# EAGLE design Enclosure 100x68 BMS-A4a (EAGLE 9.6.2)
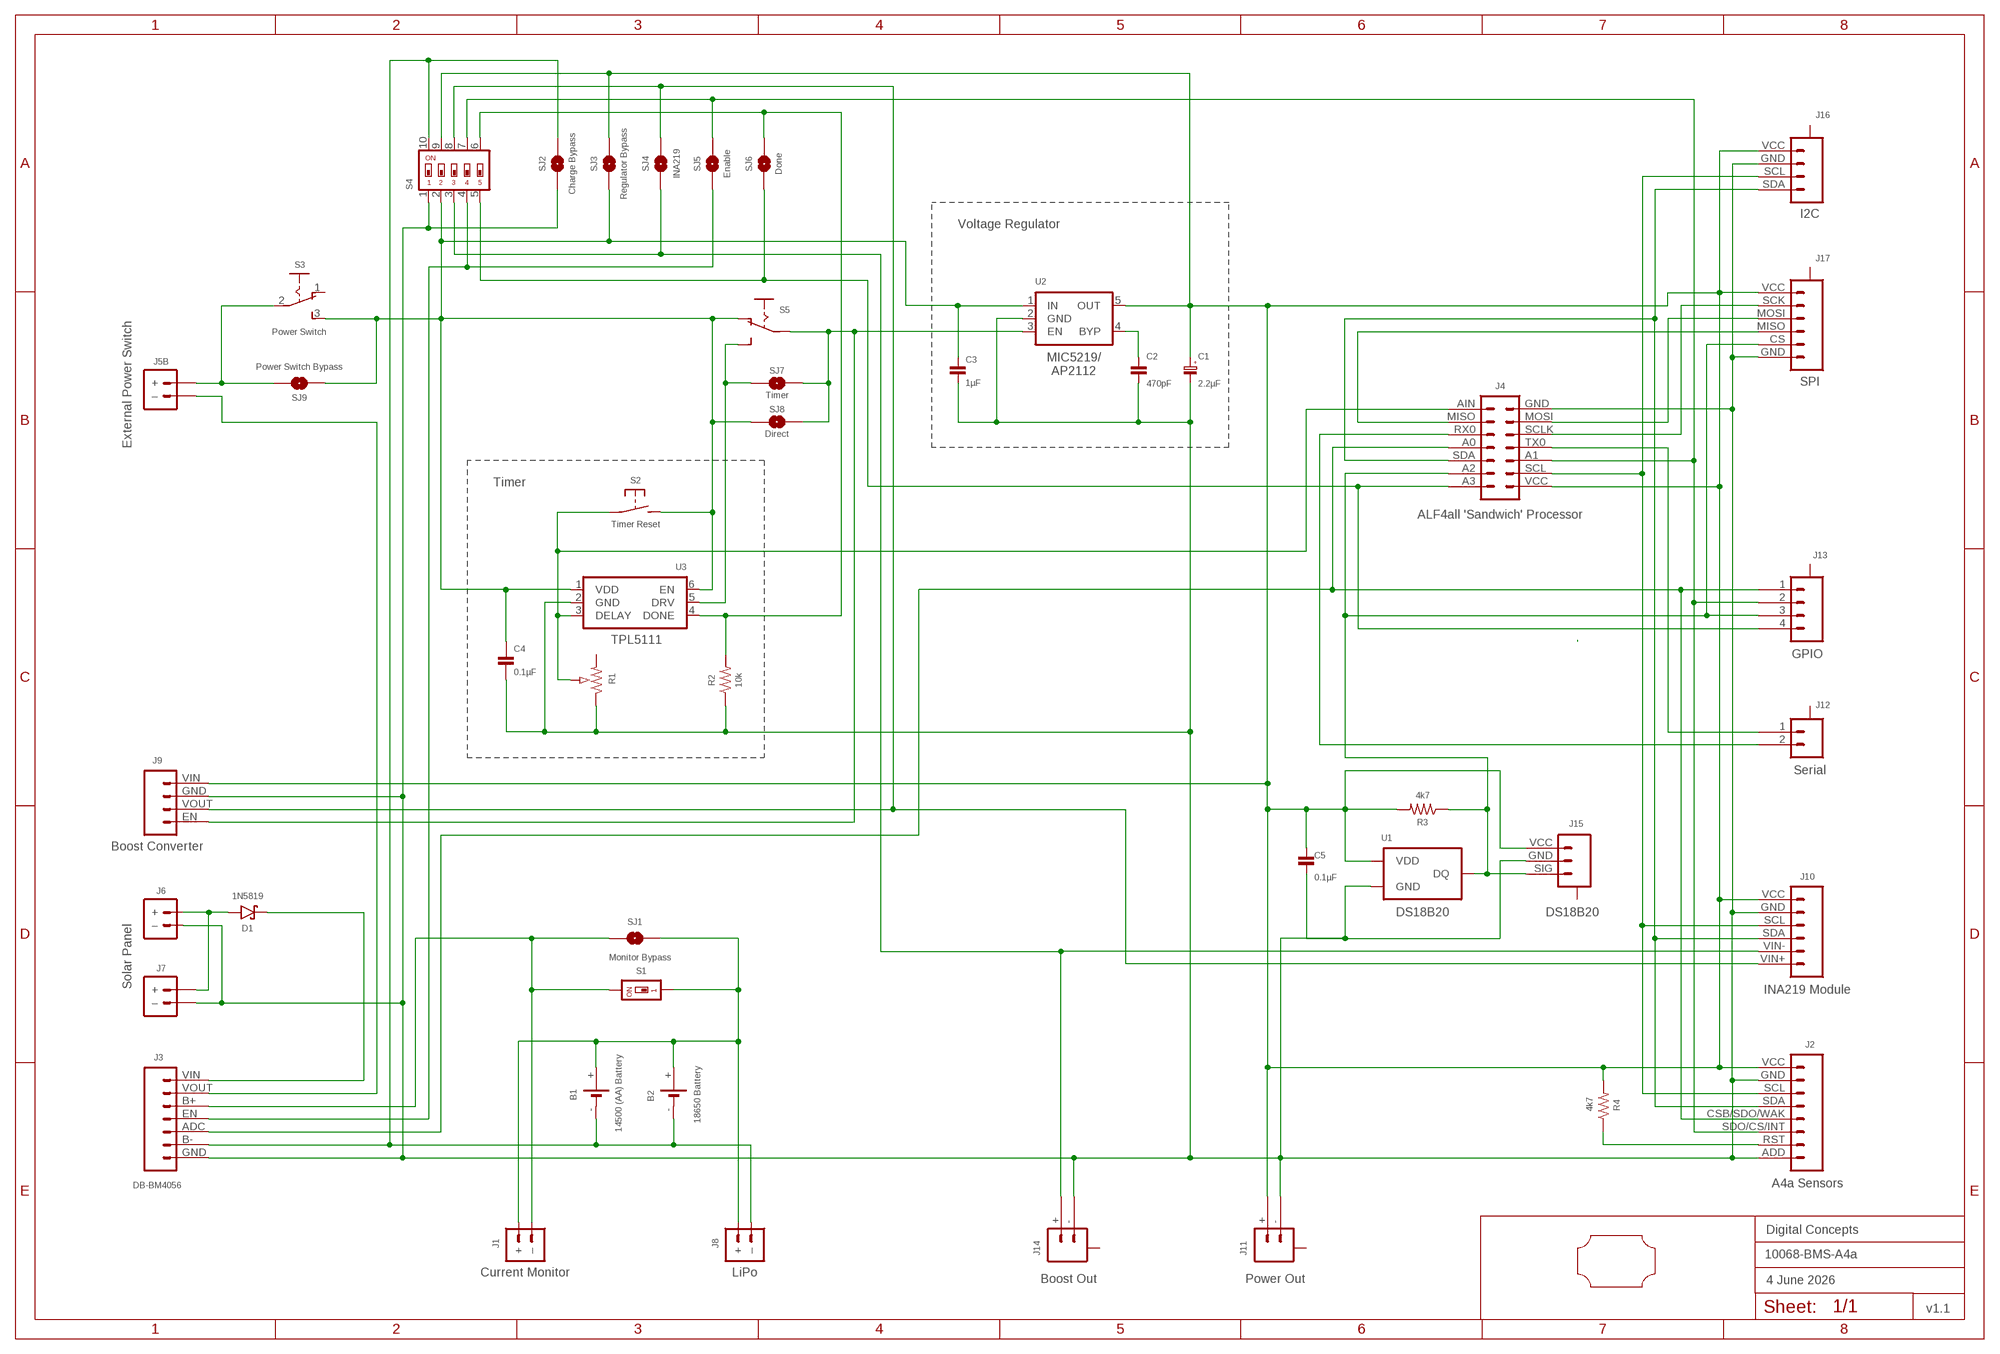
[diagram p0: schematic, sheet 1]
FRAME2 (A3L-LOC): DATE: 4 June 2026; OWNER: Digital Concepts; TITLE: 10068-BMS-A4a; VERSION: v1.1

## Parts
B1  14500 (AA) Battery  BATTERY-HOLDER-14500(AA)  [BATTERY-14500]
B2  18650 Battery  BATTERY-HOLDER-18650  [BATTERY-18650]
C1  2.2µF  CAPACITOR-1206-TANTALUM  [C1206-POLARISED]
C2  470pF  CAPACITOR-0805  [C0805]
C3  1µF  CAPACITOR-0805  [C0805]
C4  0.1µF  CAPACITOR  [C0805@1]
C5  0.1µF  CAPACITOR-0805  [C0805]
D1  1N5819  DIODE-SCHOTTKY-1N5819  [SOD-123]
J1  Current Monitor  JST-PH2.0-2-MALE-HORIZONTALJST-PTH-2  [JST-PH2.0-2-HORIZONTAL]
J2  A4a Sensors  HEADER-1X8-SENSOR  [CONN_08-SENSOR]
J3  DB-BM4056  HEADER-1X7-BCS  [CONN_07-BCS]
J4  ALF4all 'Sandwich' Processor  ALF4ALL-PROCESSOR-BOARD  [ALF4ALL-PROCESSOR-BOARD]
J5B  External Power Switch  JST-PH2.0-2-DUAL-POWERJST-PTH-2  [JST-PH2.0-2-DUAL-POWER]
J6  Solar Panel  JST-PH2.0-2-VERTICAL  [JST-PH2.0-2-VERTICAL=POWER]
J7  JST-PH2.0-2-HORIZONTAL-POWERJST-PTH-2  [JST-PH2.0-2-HORIZONTAL-POWER@1]
J8  LiPo  JST-PH2.0-2-MALE-HORIZONTALJST-PTH-2  [JST-PH2.0-2-HORIZONTAL]
J9  Boost Converter  HEADER-1X4-BOOST  [CONN_04-BOOST]
J10  INA219 Module  INA219-I2C-MODULE  [CONN_06-INA219]
J11  Power Out  JST-SH1.0-2-SMD-HORIZONTAL-POWER  [JST-SH1.0-2-SMD-HORIZONTAL-POWER]
J12  Serial  JST-SH1.0-2-SMD-HORIZONTAL  [JST-SH1.0-2-SMD-HORIZONTAL]
J13  GPIO  JST-SH1.0-4-SMD-HORIZONTAL  [JST-SH1.0-4-SMD-HORIZONTAL]
J14  Boost Out  JST-SH1.0-2-SMD-HORIZONTAL-POWER  [JST-SH1.0-2-SMD-HORIZONTAL-POWER]
J15  DS18B20  JST-SH1.0-3-SMD-HORIZONTAL-SIG  [JST-SH1.0-3-SMD-HORIZONTAL-SIG]
J16  I2C  JST-SH1.0-4-SMD-HORIZONTAL-I2C  [JST-SH1.0-4-SMD-HORIZONTAL-I2C]
J17  SPI  JST-SH1.0-6-SMD-HORIZONTAL-SPI  [JST-SH1.0-6-SMD-HORIZONTAL-SPI]
R1  RESISTOR-TRIMM-BAOTER-V-US  [RTRIM3296]
R2  10k  RESISTORR0805  [R0805]
R3  4k7  RESISTORR0805  [R0805]
R4  4k7  RESISTORR0805  [R0805]
S1  Monitor Bypass  SWITCH-DIP-SWS001-VIA-1  [SMD-001-VIA-1]
S2  Timer Reset  SWITCH-MOMENTARY-2-PIN-VIA-1  [SWITCH-2-PAD-VIA-1]
S3  Power Switch  SWITCH-SLIDE-SPDT  [SWITCH-SPDT-PTH]
S4  SWITCH-DIP-SWS005  [SMD-005]
S5  SWITCH-SLIDE-SPDT-SMT  [SWITCH-SPDT-SMT]
SJ1  Monitor Bypass  SJ  [SJ]
SJ2  Charge Bypass  SJ  [SJ]
SJ3  Regulator Bypass  SJ-V-12  [SJ-VIA-12]
SJ4  INA219  SJ  [SJ]
SJ5  Enable  SJ-V-1  [SJ-VIA-1]
SJ6  Done  SJ-V-1  [SJ-VIA-1]
SJ7  Timer  SJ-V-2  [SJ-VIA-2]
SJ8  Direct  SJ  [SJ]
SJ9  Power Switch Bypass  SJ  [SJ]
U1  DS18B20  THERMOMETER-DS18B20  [TO-92]
U2  MIC5219  [SOT-23-5]
U3  TPL5111  TPL5111DDCR  [SOT-23-6]
U$1  PCB-OUTLINE-100X68-CUT  [PROTO-34X22-OUTLINE-CUT]

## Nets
A0: J2.CSB/SDO/WAK J3.ADC J4.A0 J13.1
A1: J2.SDO/CS/INT J4.A1 J13.2 S4.7 SJ5.1 SJ5.1@V
A2: J4.A2 J13.3 J15.SIG J17.CS R3.1 U1.2(DQ)
A3: J4.A3 J13.4 S4.5 SJ6.2
AIN: J4.AIN R1.2(S) S2.1(P) S2.1@VIA(P) U3.3(DELAY)
B+: B1.+ B2.+ J1.+ J8.+ S1.1 S1.1@VIA SJ1.1
B-: B1.- B2.- J3.B- J8.-(–) S4.10 SJ2.2
BOOST-VOUT: J9.VOUT J10.VIN+ S4.8 SJ4.2
CHARGE-VOUT: J3.VOUT J5B.-(–)
GND: C1.2(-) C2.2 C3.2 C4.1 C5.2 J2.ADD J2.GND J3.GND J4.GND J6.-(–) J7.-(–) J9.GND J10.GND J11.- J14.- J15.GND J16.GND J17.GND R1.1(A) R2.1 S4.1 SJ2.1 U1.1(GND) U2.2(GND) U3.2(GND)
I-B+: J1.-(–) J3.B+ S1.2 SJ1.2
MISO: J4.MISO J17.MISO
MOSI: J4.MOSI J17.MOSI
N$1: C3.1 C4.2 S2.2(S) S3.3(S) S4.2 S5.1(O) SJ3.2 SJ3.2@V SJ8.2 SJ9.1 U2.1(IN) U3.1(VDD) U3.6(EN)
N$2: J9.EN S5.2(P) SJ7.1 SJ8.1 U2.3(EN)
N$3: C2.1 U2.4(BYP)
N$4: R2.2 S4.6 SJ6.1 SJ6.1@V U3.4(DONE)
N$5: J3.EN S4.4 SJ5.2
N$6: J5B.+ S3.2(P) SJ9.2
N$7: D1.A J6.+ J7.+
N$8: D1.C J3.VIN
N$9: S5.3(S) SJ7.2 SJ7.2@V U3.5(DRV)
RST: J2.RST R4.1
RXO: J4.RX0 J12.2
SCK: J4.SCLK J17.SCK
SCL: J2.SCL J4.SCL J10.SCL J16.SCL
SDA: J2.SDA J4.SDA J10.SDA J16.SDA
TXO: J4.TX0 J12.1
VCC: C1.1(+) C5.1 J2.VCC J4.VCC J9.VIN J10.VCC J11.+ J15.VCC J16.VCC J17.VCC R3.2 R4.2 S4.9 SJ3.1 SJ3.1@V U1.3(VDD) U2.5(OUT)
VDD: J10.VIN- J14.+ S4.3 SJ4.1
Unconnected: J11.A@1(A) J11.A@2(A) J12.A@1(A) J12.A@2(A) J13.A@1(A) J13.A@4(A) J14.A@1(A) J14.A@2(A) J15.A@1(A) J15.A@3(A) J16.A@1(A) J16.A@4(A) J17.A@1(A) J17.A@6(A) R1.3(E) S3.1(O)

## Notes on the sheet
- Voltage Regulator
- MIC5219/
  AP2112
- Timer

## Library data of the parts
B1 = digitalconcepts:BATTERY-HOLDER-14500(AA): 14500 (AA) battery holder
B2 = digitalconcepts:BATTERY-HOLDER-18650: 18650 Battery Holder
C1 = digitalconcepts:CAPACITOR-1206-TANTALUM: Capacitor 1206 Tantalum
C2 C3 C5 = digitalconcepts:CAPACITOR-0805: 0805 Capacitor
C4 = digitalconcepts:CAPACITOR: 0805 Capacitor
D1 = digitalconcepts:DIODE-SCHOTTKY-1N5819: 1N5819 Schottky Diode SOD-123
J1 J8 = digitalconcepts:JST-PH2.0-2-MALE-HORIZONTAL: PH2.0 2P Right Angle PCB Connector; PROD_ID: CONN-09863; SKU: PRT-09914
J2 = digitalconcepts:HEADER-1X8-SENSOR: IoT Sensors 1x8 Pin Header for 'Sandwich' IoT Sensors
J3 = digitalconcepts:HEADER-1X7-BCS: Single Row 7-Pin Header BCS Pin labels
J4 = digitalconcepts:ALF4ALL-PROCESSOR-BOARD: ALF4all 'Sandwixh' Processor 2x7 Pin Header and earthed 1x1 locator pins for ALF4all 'Sandwich' Processor/RFM95W PCBs
J5B = digitalconcepts:JST-PH2.0-2-DUAL-POWER: JST PH2.0 2P PTH Dual-Side Connector (Power); PROD_ID: CONN-09863; SKU: PRT-09914
J6 = digitalconcepts:JST-PH2.0-2-VERTICAL: PH2.0 2P PCB Connector
J7 = digitalconcepts:JST-PH2.0-2-HORIZONTAL-POWER: PH2.0 2P Right Angle PCB Connector; PROD_ID: CONN-09863; SKU: PRT-09914
J9 = digitalconcepts:HEADER-1X4-BOOST: Boost Converter Module 4-Pin Header
J10 = digitalconcepts:INA219-I2C-MODULE: INA219 I2C Module
J11 J14 = digitalconcepts:JST-SH1.0-2-SMD-HORIZONTAL-POWER: JST SH1.0 2P SMD Horizontal Connector with Power Labels
J12 = digitalconcepts:JST-SH1.0-2-SMD-HORIZONTAL: JST SH1.0 2P SMD Horizontal Connector
J13 = digitalconcepts:JST-SH1.0-4-SMD-HORIZONTAL: JST SH1.0 4P SMD horizontal connector
J15 = digitalconcepts:JST-SH1.0-3-SMD-HORIZONTAL-SIG: JST SH1.0 3P SMD Horizontal Connector with Signal
J16 = digitalconcepts:JST-SH1.0-4-SMD-HORIZONTAL-I2C: JST SH1.0 4P SMD I2C horizontal connector
J17 = digitalconcepts:JST-SH1.0-6-SMD-HORIZONTAL-SPI: JST SH1.0 6P SMD SPI horizontal connector
R1 = digitalconcepts:RESISTOR-TRIMM-BAOTER-V-US: Trimm Resistor - Vertical BAOTER
R2-R4 = digitalconcepts:RESISTOR: Resistor; SPICEPREFIX: R
S1 = digitalconcepts:SWITCH-DIP-SWS001-VIA-1: SMD Dip Switch 1 pol.
S2 = digitalconcepts:SWITCH-MOMENTARY-2-PIN-VIA-1: 2 Pin Momentary Switch
S3 = digitalconcepts:SWITCH-SLIDE-SPDT: Mini Sliding Switch SPDT
S4 = digitalconcepts:SWITCH-DIP-SWS005: SMD Dip Switch 5 pol.
S5 = digitalconcepts:SWITCH-SLIDE-SPDT-SMT: Mini Sliding Switch SPDT SMT
SJ1 SJ2 SJ4 SJ8 SJ9 = digitalconcepts:SJ: Solder Jumper
SJ3 = digitalconcepts:SJ-V-12: Solder Jumper with Pad Vias
SJ5 SJ6 = digitalconcepts:SJ-V-1: Solder Jumper with single Pad Via
SJ7 = digitalconcepts:SJ-V-2: Solder Jumper with Pad Vias
U1 = digitalconcepts:THERMOMETER-DS18B20: Digital Thermometer -55C-125C TO92-3; AVAILABILITY: Bad; DESCRIPTION: Temperature Sensor Digital, Local -55°C ~ 125°C 12 b 8-uMAX; MF: Maxim Integrated; MP: DS18B20; PACKAGE: TO-92 Maxim Integrated; PRICE: None
U2 = digitalconcepts:MIC5219: Microchip LDO Linear Voltage Regulator; OC_FARNELL: unknown; OC_NEWARK: unknown
U3 = digitalconcepts:TPL5111DDCR: TPL5111 Nano-Power System Timer
U$1 = digitalconcepts:PCB-OUTLINE-100X68-CUT: PCB outline for 100 x 68 enclosure with long side cut-out

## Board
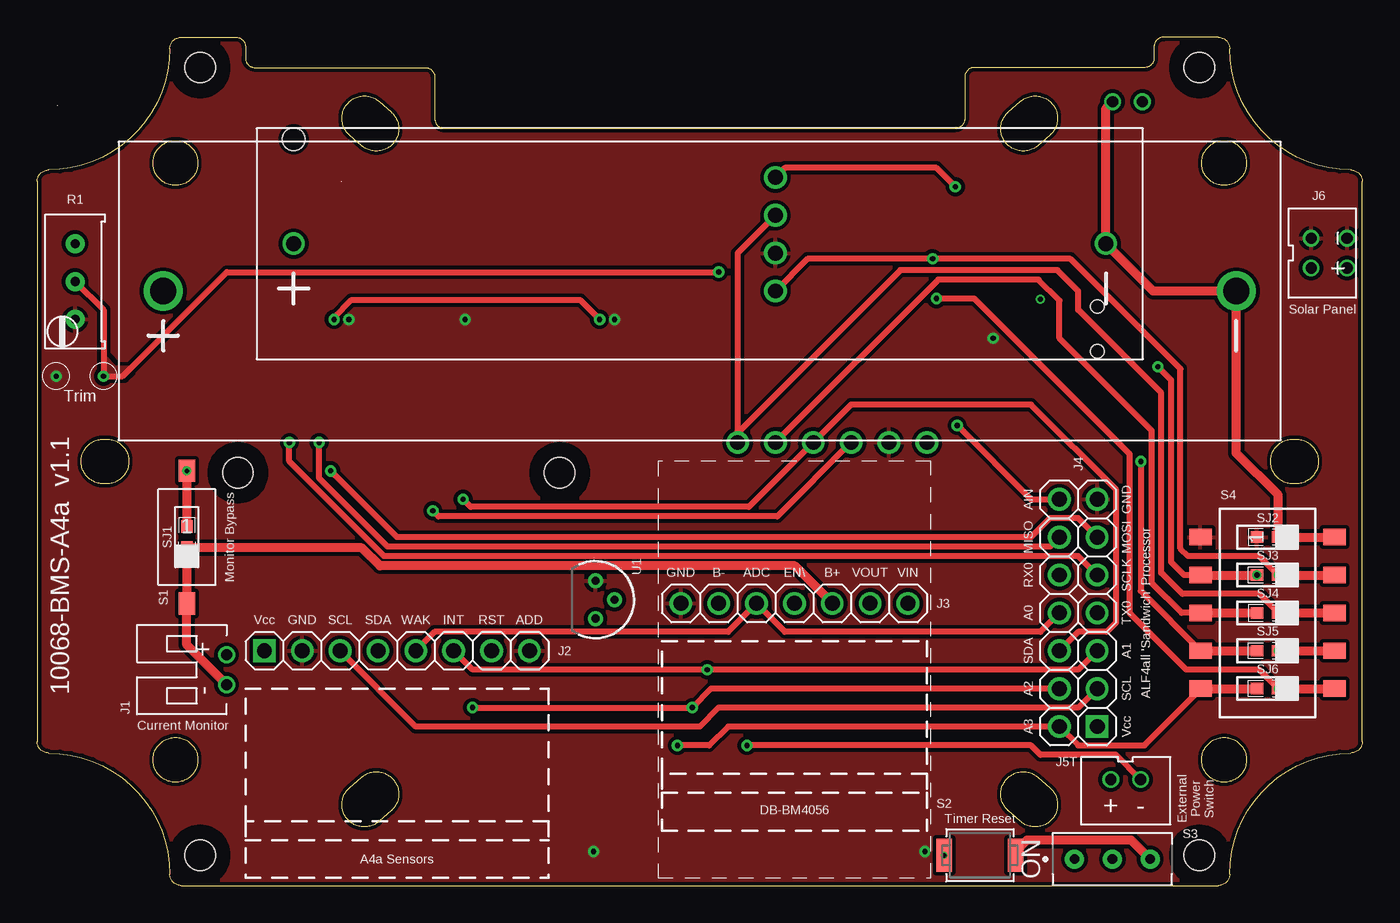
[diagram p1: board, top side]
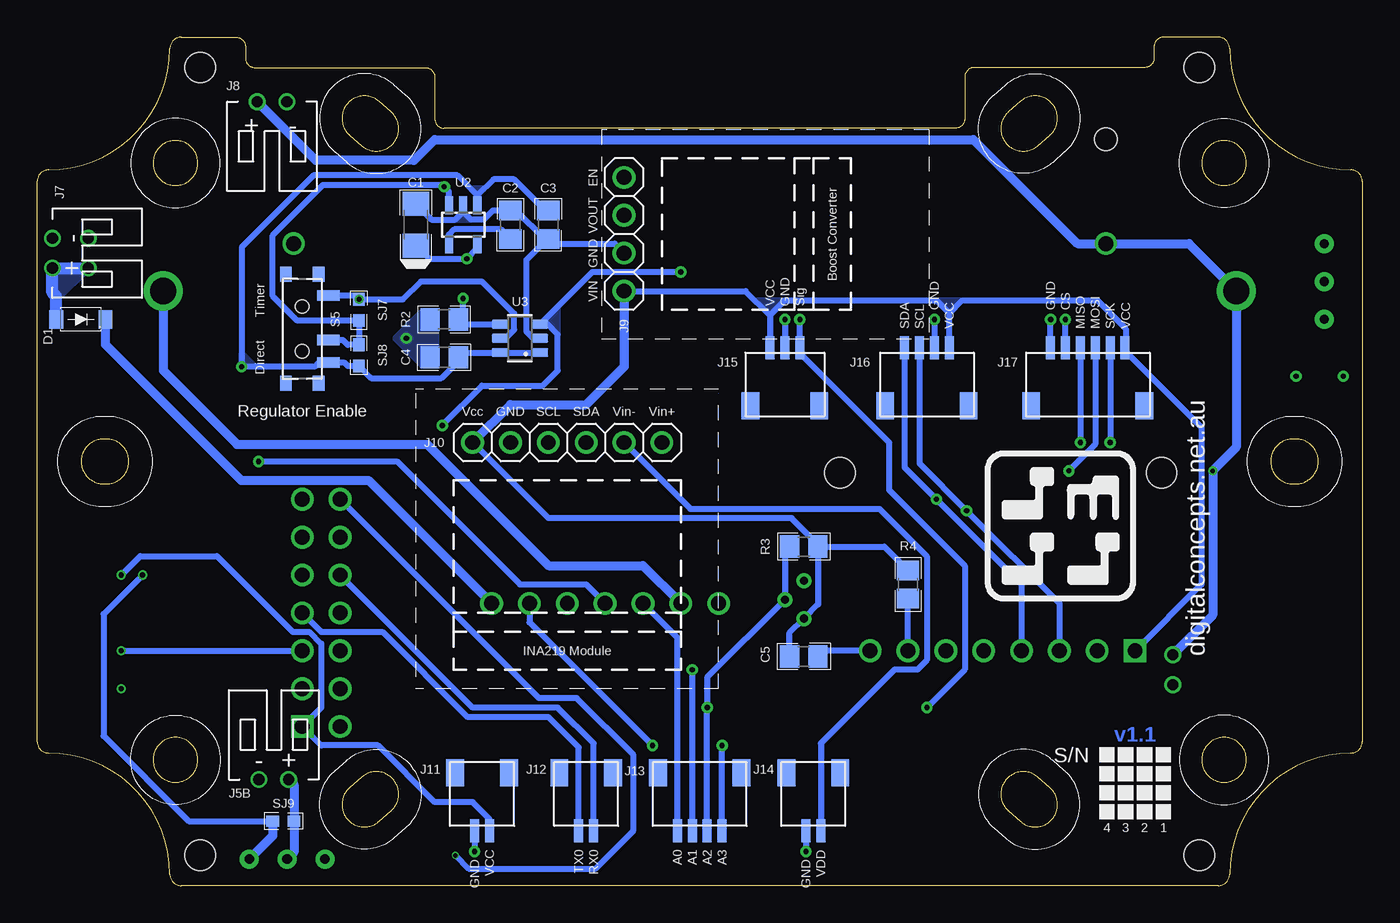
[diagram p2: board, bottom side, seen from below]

Size 88.9 x 56.9 mm. Coordinates in mm from the lower left corner, seen from the top.
Copper layers (1*16): Top 0.035mm / dielectric 1.5mm / Bottom 0.035mm
Design rules "default *": minimum track width 6mil, minimum drill 0.3mm, track to track 6mil, track to pad 6mil, pad to pad 6mil, via to via 6mil, smd to smd 6mil, copper to edge 6mil, drill to drill 6mil, minimum pad ring 1mil, minimum via ring 8mil, stop-mask expansion 4mil, vias tented up to drill 0mil, thermal gap 10mil
Holes 2.03 mm at 13.46,27.69 35.05,27.69

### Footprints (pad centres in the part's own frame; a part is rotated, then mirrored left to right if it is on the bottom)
BATTERY-14500 = drill 1: + -27.25,0; - 27.25,0 | hole 1.524: -27.25,7
BATTERY-18650 = drill 1.75: + -36,0; - 36,0
C1206-POLARISED = smd 1.6 x 1.8: 1 -1.4,0; 2 1.4,0
C0805 = smd 1.3 x 1.5: 1 -0.95,0; 2 0.95,0
C0805@1 = smd 1.3 x 1.5: 1 -0.95,0; 2 0.95,0
SOD-123 = smd 0.91 x 1.22: A -1.65,0; C 1.65,0
JST-PH2.0-2-HORIZONTAL = drill 0.75: + 1,0; - -1,0
CONN_08-SENSOR = drill 1 pad 1.524: ADD 17.78,0; CSB/SDO/WAK 10.16,0; GND 2.54,0; RST 15.24,0; SCL 5.08,0; SDA 7.62,0; SDO/CS/INT 12.7,0 | drill 1 pad 1.524 square: VCC 0,0
CONN_07-BCS = drill 1 pad 1.524: ADC 5.08,0; B+ 10.16,0; B- 2.54,0; EN 7.62,0; GND 0,0; VIN 15.24,0; VOUT 12.7,0
ALF4ALL-PROCESSOR-BOARD = drill 1 pad 1.524: A0 7.62,2.54; A1 5.08,0; A2 2.54,2.54; A3 0,2.54; AIN 15.24,2.54; GND 15.24,0; MISO 12.7,2.54; MOSI 12.7,0; RX0 10.16,2.54; SCL 2.54,0; SCLK 10.16,0; SDA 5.08,2.54; TX0 7.62,0 | drill 1 pad 1.524 square: VCC 0,0
JST-PH2.0-2-DUAL-POWER = drill 0.75: + 1,0; - -1,0
JST-PH2.0-2-VERTICAL=POWER = drill 0.75: + -1,0; - 1,0
JST-PH2.0-2-HORIZONTAL-POWER@1 = drill 0.75: + 1,0; - -1,0
CONN_04-BOOST = drill 1 pad 1.524: EN 0,0; GND 5.08,0; VIN 7.62,0; VOUT 2.54,0
CONN_06-INA219 = drill 1 pad 1.524: GND 2.54,0; SCL 5.08,0; SDA 7.62,0; VCC 0,0; VIN+ 12.7,0; VIN- 10.16,0
JST-SH1.0-2-SMD-HORIZONTAL-POWER = smd 0.6 x 1.55: + -0.5,2.54; - 0.5,2.54 | smd 1.2 x 1.8: A@1 1.8,-1.335; A@2 -1.8,-1.335
JST-SH1.0-2-SMD-HORIZONTAL = smd 0.6 x 1.55: 1 0.5,2.54; 2 -0.5,2.54 | smd 1.2 x 1.8: A@1 1.8,-1.335; A@2 -1.8,-1.335
JST-SH1.0-4-SMD-HORIZONTAL = smd 0.6 x 1.55: 1 1.5,2.54; 2 0.5,2.54; 3 -0.5,2.54; 4 -1.5,2.54 | smd 1.2 x 1.8: A@1 2.8,-1.335; A@4 -2.8,-1.335
JST-SH1.0-3-SMD-HORIZONTAL-SIG = smd 1.2 x 1.8: A@1 2.3,-1.335; A@3 -2.3,-1.335 | smd 0.6 x 1.55: GND 0,2.54; SIG 1,2.54; VCC -1,2.54
JST-SH1.0-4-SMD-HORIZONTAL-I2C = smd 1.2 x 1.8: A@1 2.8,-1.335; A@4 -2.8,-1.335 | smd 0.6 x 1.55: GND 0.5,2.54; SCL -0.5,2.54; SDA -1.5,2.54; VCC 1.5,2.54
JST-SH1.0-6-SMD-HORIZONTAL-SPI = smd 1.2 x 1.8: A@1 3.8,-1.335; A@6 -3.8,-1.335 | smd 0.6 x 1.55: CS -1.5,2.54; GND -2.5,2.54; MISO -0.5,2.54; MOSI 0.5,2.54; SCK 1.5,2.54; VCC 2.5,2.54
RTRIM3296 = drill 0.61 pad 1.27: 1 0,-2.54; 2 0,0; 3 0,2.54
R0805 = smd 1.3 x 1.5: 1 -0.95,0; 2 0.95,0
SMD-001-VIA-1 = smd 1.1 x 1.5: 1 0,-4.45; 2 0,4.45 | drill 0.3 pad 0.61: 1@VIA 0,-4.45
SWITCH-2-PAD-VIA-1 = smd 1.067 x 2.184: 1 -2.4,0; 2 2.4,0 | drill 0.3: 1@VIA -2.4,0
SWITCH-SPDT-PTH = drill 0.65 pad 1.27: 1 -2.54,0; 2 0,0; 3 2.54,0
SMD-005 = smd 1.1 x 1.5: 1 -5.08,-4.5; 2 -2.54,-4.5; 3 0,-4.5; 4 2.54,-4.5; 5 5.08,-4.5; 6 5.08,4.5; 7 2.54,4.5; 8 0,4.5; 9 -2.54,4.5; 10 -5.08,4.5
SWITCH-SPDT-SMT = smd 0.7 x 1.5: 1 2.25,1.75; 2 0.75,1.75; 3 -2.25,1.75 | smd 1 x 0.8: GND@1 3.65,-1.1; GND@2 3.65,1.1; GND@3 -3.65,1.1; GND@4 -3.65,-1.1 | hole 0.9: -1.5,0; 1.5,0
SJ = smd 0.864 x 0.762: 1 -0.711,0; 2 0.711,0
SJ-VIA-12 = smd 0.864 x 0.762: 1 -0.711,0; 2 0.711,0 | drill 0.35 pad 0.61: 1@V -0.711,0; 2@V 0.711,0
SJ-VIA-1 = smd 0.864 x 0.762: 1 -0.711,0; 2 0.711,0 | drill 0.35 pad 0.61: 1@V -0.711,0
SJ-VIA-2 = smd 0.864 x 0.762: 1 -0.711,0; 2 0.711,0 | drill 0.35 pad 0.61: 2@V 0.711,0
TO-92 = drill 0.55 pad 1.016: 1 -1.27,0; 2 0,1.27; 3 1.27,0
SOT-23-5 = smd 0.55 x 1.2: 1 -0.95,-1.3; 2 0,-1.3; 3 0.95,-1.3; 4 0.95,1.3; 5 -0.95,1.3
SOT-23-6 = smd 1.1 x 0.6: 1 -1.35,0.95; 2 -1.35,0; 3 -1.35,-0.95; 4 1.35,-0.95; 5 1.35,0; 6 1.35,0.95
PROTO-34X22-OUTLINE-CUT = hole 2.032: -33.528,26.416; 33.528,26.416; 33.528,-26.416; -33.528,-26.416

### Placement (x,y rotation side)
B1  44.45,43.05 0 top
B2  44.45,39.88 0 top
C1  63.5,44.32 90 bottom
C2  57.15,44.32 90 bottom
C3  54.61,44.32 270 bottom
C4  61.59,35.43 0 bottom
C5  37.47,15.37 0 bottom
D1  85.98,37.97 0 bottom
J1  12.7,14.48 90 top
J2  15.24,15.75 0 top
J3  43.18,18.92 0 top
J4  71.12,10.67 90 top
J5B  73.03,7.11 0 bottom
J6  85.47,42.42 90 top
J7  87.88,42.42 270 bottom
J8  73.15,52.58 180 bottom
J9  49.53,47.5 270 bottom
J10  59.69,29.72 0 bottom
J11  59.06,6.22 180 bottom
J12  52.07,6.22 180 bottom
J13  44.45,6.22 180 bottom
J14  36.83,6.22 180 bottom
J15  38.73,33.53 0 bottom
J16  29.21,33.53 0 bottom
J17  18.42,33.53 0 bottom
R1  2.54,40.51 0 top
R2  61.59,37.97 0 bottom
R3  37.47,22.73 0 bottom
R4  30.48,20.19 90 bottom
S1  10.03,23.37 180 top
S2  63.25,2.03 0 top
S3  72.14,1.78 0 top
S4  82.55,18.29 270 top
S5  71.12,37.34 270 bottom
SJ1  10.03,23.37 270 top
SJ2  82.55,23.37 0 top
SJ3  82.55,20.83 180 top
SJ4  82.55,18.29 0 top
SJ5  82.55,15.75 180 top
SJ6  82.55,13.21 180 top
SJ7  67.31,38.61 90 bottom
SJ8  67.31,35.56 270 bottom
SJ9  72.39,4.32 0 bottom
U1  37.47,19.18 270 top
U2  60.33,44.32 180 bottom
U3  56.52,36.7 180 bottom
U$1  44.45,28.45 0 top

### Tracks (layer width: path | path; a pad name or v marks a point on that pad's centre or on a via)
$X0
  cutout Bottom: 10.92,56.9 arc180 10.92,52.83 arc180
$X1
  cutout Bottom: 77.98,56.9 arc180 77.98,52.83 arc180
$X2
  cutout Bottom: 77.98,4.06 arc180 77.98,0 arc180
$X3
  cutout Bottom: 10.92,4.06 arc180 10.92,0 arc180
$X4
  cutout Top: 10.92,56.9 arc180 10.92,52.83 arc180
$X5
  cutout Top: 77.98,56.9 arc180 77.98,52.83 arc180
$X6
  cutout Top: 77.98,4.06 arc180 77.98,0 arc180
$X7
  cutout Top: 10.92,4.06 arc180 10.92,0 arc180
$X8
  cutout Bottom: 13.46,29.72 arc180 13.46,25.65 arc180
$X9
  cutout Top: 35.05,29.72 arc180 35.05,25.65 arc180
$X10
  cutout Top: 13.46,29.72 arc180 13.46,25.65 arc180
$X11
  cutout Bottom: 35.05,29.72 arc180 35.05,25.65 arc180
A0
  Top 0.406: J4.A0 67.31,17.02 50.16,17.02 J3.ADC 46.36,17.02 26.67,17.02 J2.CSB/SDO/WAK
  Bottom 0.406: J3.ADC 45.95,16.61 J13.1
A1  (via drill 0.35)
  Top 0.406: J4.A1 69.85,14.48 v44.95,14.48 29.21,14.48 J2.SDO/CS/INT
  Top 0.61: SJ5.1@V S4.7
  Bottom 0.406: SJ5.1@V J4.A1 | J13.2 v44.95,14.48
A2  (via drill 0.35)
  Top 0.406: J4.A2 45.22,13.21 v43.95,11.94 v29.21,11.94 | v37.73,37.97 36.47,39.24 21.06,39.24 19.92,38.1 v19.92,37.97
  Bottom 0.406: R3.1 38.73,22.41 U1.2 43.95,13.96 v43.95,11.94 J13.3 | J17.CS v19.92,37.97 | v37.73,37.97 J15.SIG 37.73,35.7 31.75,29.72 31.75,26.54 26.67,21.46 26.67,14.48 v29.21,11.94
A3  (via drill 0.35)
  Top 0.406: v42.95,9.4 45.09,9.4 46.36,10.67 J4.A3 69.85,9.4 74.3,9.4 78.05,13.15 S4.5
  Top 0.61: S4.5 SJ6.2
  Bottom 0.406: J13.4 v42.95,9.4
AIN  (via drill 0.35)
  Top 0.406: J4.AIN 66.67,25.91 v61.72,30.86 | R1.2 4.45,38.61 v4.45,34.16 5.73,34.16 12.71,41.15 v45.72,41.15
  Bottom 0.406: v61.72,30.86 59.06,33.53 54.99,33.53 53.98,34.54 53.98,36.96 54.67,37.65 U3.3 51.67,41.15 v45.72,41.15 | S2.1@VIA 59.96,1.14 51.44,1.14 48.9,3.68 48.9,8.76 52.7,12.57 55.25,12.57 J4.AIN
  pour Bottom (no thermals): 54.86,37.85 53.98,38.73 53.98,36.96
  pour Top (no thermals): 4.45,34.16 5.72,34.16 6.22,34.67 5.21,34.67 4.45,35.43
B+
  Top 0.61: S1.1@VIA SJ1.1
  Bottom 0.61: J1.+ 10.03,18.15 S1.1@VIA 8.45,29.4 B2.+ 11.62,43.05 B1.+ 19.11,43.05 26.09,50.04 62.23,50.04 63.63,48.64 70.22,48.64 J8.+
B-
  Top 0.61: J8.- 71.7,52.13 B1.- 74.88,39.88 B2.- 80.45,29.01 83.26,26.2 SJ2.2 S4.10
  Bottom 0.61: B2.- 80.45,34.55 75.49,29.59 62.74,29.59 54.61,21.46 48.26,21.46 J3.B-
BOOST-VOUT
  Top 0.406: J9.VOUT 46.99,42.42 J10.VIN+ 46.99,30.35 57.91,41.28 68.45,41.28 69.85,39.88 69.85,38.61 75.41,33.05 75.41,20.98 76.84,19.56 81.99,19.56 SJ4.2
  Top 0.61: SJ4.2 S4.8
CHARGE-VOUT  (via drill 0.35)
  Top 0.406: J5B.- 72.39,8.75 72.39,8.76 67.31,8.76 66.67,9.4 v47.62,9.4
  Bottom 0.406: J3.VOUT 55.88,17.65 v47.62,9.4
GND  (via drill 0.35)
  Bottom 0.406: C1.2 62.45,44.67 60.85,44.67 60.33,45.2 | 60.33,45.2 59.8,44.67 58.95,44.67 58.35,45.27 C2.2 56.77,45.27 54.87,43.37 C3.2 54.61,43.31 54.36,43.05 | U2.2 60.33,45.2 | U3.2 55.63,36.7 56.08,37.16 56.08,41.96 54.99,43.05 54.36,43.05 | 54.36,43.05 50.16,43.05 J9.GND | v38.73,37.97 J15.GND | v28.71,37.97 J16.GND | J17.GND v20.92,37.97 | J14.- v37.33,2.29 | J11.- v59.56,2.29 | J2.ADD 36.13,15.75 C5.2
  other vias: 64.14,36.7 1.27,34.16
  pour Top (isolate 0.254, rank 5): -1.06,57.55 -1.06,-0.7 89.91,-0.7 89.91,57.55
  pour Bottom (no thermals): 60.33,45.2 60.85,44.67 59.8,44.67
  pour Bottom (no thermals): 64.9,36.7 63.12,34.93 62.1,34.93 62.1,38.48 63.12,38.48
I-B+
  Top 0.61: J1.- 10.03,16.15 S1.2 SJ1.2 21.77,22.66 22.99,21.44 50.83,21.44 J3.B+
MISO  (via drill 0.35)
  Top 0.406: J4.MISO 67.95,22.73 23.5,22.73 18.92,27.31 v18.92,29.72
  Bottom 0.406: J17.MISO v18.92,29.72
MOSI  (via drill 0.35)
  Top 0.406: J4.MOSI 69.85,24.64 67.95,24.64 66.67,23.37 24.13,23.37 v19.69,27.81
  Bottom 0.406: J17.MOSI 17.92,29.58 v19.69,27.81
N$1  (via drill 0.35)
  Top 0.406: S4.2 76.96,20.83 76.07,21.71 76.07,33.91 v75.18,34.8
  Top 0.61: S2.2 65.65,2.29 66.41,3.05 73.41,3.05 S3.3 | S4.2 SJ3.2@V
  Bottom 0.406: 59.38,46.29 58.3,47.37 56.9,47.37 54.8,45.27 C3.1 | 59.38,46.29 60.71,47.62 70.36,47.62 75.18,42.8 v75.18,34.8 70.3,34.8 70,35.09 S5.1 68.31,35.09 68.07,34.85 SJ8.2 66.5,34.04 61.78,34.04 60.64,35.18 C4.2 60.85,35.75 U3.6 U3.1 | 59.38,46.29 U2.1 | SJ3.2@V 84.45,18.21 84.45,10.03 78.74,4.32 SJ9.1
  Bottom 0.61: SJ9.1 73.1,3.35 S3.3
  pour Bottom (no thermals): 58.93,46.74 59.82,46.74 59.38,46.29
  pour Bottom (no thermals): 75.18,34.8 75.18,35.69 74.3,34.8
N$2  (via drill 0.35)
  Top 0.406: v61.59,46.86 60.33,48.13 50.16,48.13 J9.EN
  Bottom 0.406: U2.3 61.28,46.54 v61.59,46.86 61.72,46.99 69.72,46.99 73.1,43.61 73.1,39.54 71.46,37.9 SJ7.1 SJ8.1 68.07,36.27 68.39,36.59 S5.2
N$3
  Bottom 0.406: U2.4 61.28,43.66 60.92,44.01 57.79,44.01 C2.1
N$4  (via drill 0.35)
  Top 0.406: v60.33,39.37 62.86,39.37 73.28,28.96 73.28,18.29 77.09,14.48 81.99,14.48 SJ6.1@V
  Top 0.61: SJ6.1@V S4.6
  Bottom 0.406: U3.4 60.33,37.65 R2.2 60.33,38.29 v60.33,39.37
N$5  (via drill 0.35)
  Top 0.406: S4.4 74.04,19.76 v74.04,28.45
  Top 0.61: S4.4 SJ5.2
  Bottom 0.406: v74.04,28.45 64.77,28.45 56.52,20.19 52.07,20.19 J3.EN
N$6
  Bottom 0.61: J5B.+ 71.68,6.77 SJ9.2 71.68,2.24 S3.2
N$7
  Bottom 0.813: D1.A 87.63,39.51 87.88,39.77 J7.+ J6.+
  pour Bottom (no thermals): 87.63,41.42 85.73,41.42 87.63,39.51
N$8
  Bottom 0.61: D1.C 84.33,36.3 75.21,27.18 66.67,27.18 J3.VIN
N$9
  Bottom 0.406: U3.5 57.48,36.7 56.9,37.29 56.9,38.35 59.06,40.51 63.18,40.51 64.37,39.32 SJ7.2@V 67.58,39.59 S5.3
RST
  Bottom 0.406: J2.RST R4.1
RXO
  Bottom 0.406: J12.2 51.57,9.53 53.98,11.94 59.69,11.94 J4.RX0
SCK  (via drill 0.35)
  Top 0.406: J4.SCLK 69.85,22.1 23.27,22.1 16.92,28.45 v16.92,29.72
  Bottom 0.406: J17.SCK v16.92,29.72
SCL  (via drill 0.35)
  Top 0.406: J4.SCL 69.85,11.94 45.72,11.94 44.45,10.67 25.4,10.67 J2.SCL | J10.SCL 49.66,24.77 26.92,24.77 v26.54,25.15
  Bottom 0.406: J16.SCL 29.71,28.31 v26.54,25.15 20.32,18.92 J2.SCL
SDA  (via drill 0.35)
  Top 0.406: v28.58,25.91 29.08,25.4 47.75,25.4 J10.SDA 54.61,32.26 66.67,32.26 72.39,26.54 72.39,17.65 71.75,17.02 69.85,17.02 J4.SDA
  Bottom 0.406: J16.SDA 30.71,28.04 v28.58,25.91 22.86,20.19 J2.SDA
TXO
  Bottom 0.406: J12.1 52.57,9.26 54.61,11.3 60.01,11.3 65.73,17.02 69.85,17.02 J4.TX0
VCC  (via drill 0.35)
  Top 0.406: J9.VIN 51.69,42.04 v60.07,42.04 69.32,42.04 76.71,34.65 76.71,22.61 77.22,22.1 81.99,22.1 SJ3.1@V
  Top 0.61: SJ3.1@V S4.9
  Bottom 0.406: C1.1 62.61,42.04 v60.07,42.04 59.38,42.73 U2.5 | C5.1 38.41,16.96 U1.3 36.52,18.86 R3.2 | J2.VCC 10.8,20.19 10.8,30.73 15.92,35.85 J17.VCC 15.88,36.07 15.88,37.34 17.78,39.24 26.85,39.24 27.71,38.38 | J11.+ 58.55,4.45 59.69,5.59 62.23,5.59 66.04,9.4 69.85,9.4 J4.VCC 69.85,11.94 69.85,16.23 70.64,17.02 71.75,17.02 76.84,22.1 81.99,22.1 SJ3.1@V | J16.VCC 27.71,38.38 | 39.73,38.24 38.73,39.24 28.58,39.24 27.71,38.38 | 39.73,38.24 41.37,39.88 J9.VIN | R3.2 36.52,22.86 38.29,24.64 54.61,24.64 J10.VCC | 39.73,38.24 J15.VCC | R3.2 32.07,22.73 R4.2
  Bottom 0.61: J10.VCC 57.15,32.26 52.07,32.26 49.53,34.8 J9.VIN
  pour Bottom (no thermals): 39.73,38.24 40.73,39.24 38.73,39.24
  pour Bottom (no thermals): 27.71,38.38 28.58,39.24 26.85,39.24
VDD
  Top 0.406: S4.3 76.78,18.29 74.78,20.29 74.78,30.51 68.58,36.7 68.58,39.24 67.18,40.64 60.45,40.64 J10.VIN-
  Top 0.61: S4.3 SJ4.1
  Bottom 0.406: J14.+ 36.33,9.53 31.39,14.48 29.84,14.48 29.21,15.11 29.21,22.1 32.39,25.27 45.09,25.27 J10.VIN-

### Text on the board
Bottom: v1.1
tPlace: AIN | GND | MISO | MOSI | 10068-BMS-A4a v1.1 | GND | B- | ADC | EN\ | B+ | VOUT | VIN | RX0 | SCLK | A0 | TX0 | Vcc | GND | SCL | SDA | WAK | INT | RST | ADD | SDA | A1 | A2 | SCL | A3 | Vcc
bPlace: EN | VOUT | GND | VIN | Vin+ | Vin- | SDA | SCL | GND | Vcc | digitalconcepts.net.au | S/N | 1 | 2 | 3 | 4
tNames: Trim | Monitor Bypass | J5T | External / Power / Switch | ON
bNames: CS | GND | GND | Sig | GND | VCC | Timer | VCC | SCK | MOSI | MISO | VCC | SCL | SDA | Direct | Regulator Enable | VDD | GND | A3 | A2 | A1 | A0 | RX0 | TX0 | VCC | GND
bValues: MIC5219 / AP2112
